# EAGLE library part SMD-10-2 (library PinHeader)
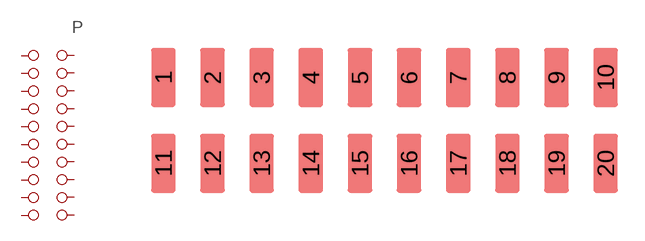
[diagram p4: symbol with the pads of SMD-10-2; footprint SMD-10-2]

Designator prefix P

## SMD-10-2  [SMD-10-2]
1  1  pas
2  2  pas
3  3  pas
4  4  pas
5  5  pas
6  6  pas
7  7  pas
8  8  pas
9  9  pas
10  10  pas
11  11  pas
12  12  pas
13  13  pas
14  14  pas
15  15  pas
16  16  pas
17  17  pas
18  18  pas
19  19  pas
20  20  pas

## Footprint SMD-10-2 (pad centres in mm)
smd 1.27 x 3.048: 1 -11.43,2.223; 2 -8.89,2.223; 3 -6.35,2.223; 4 -3.81,2.223; 5 -1.27,2.223; 6 1.27,2.223; 7 3.81,2.223; 8 6.35,2.223; 9 8.89,2.223; 10 11.43,2.223; 11 -11.43,-2.223; 12 -8.89,-2.223; 13 -6.35,-2.223; 14 -3.81,-2.223; 15 -1.27,-2.223; 16 1.27,-2.223; 17 3.81,-2.223; 18 6.35,-2.223; 19 8.89,-2.223; 20 11.43,-2.223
